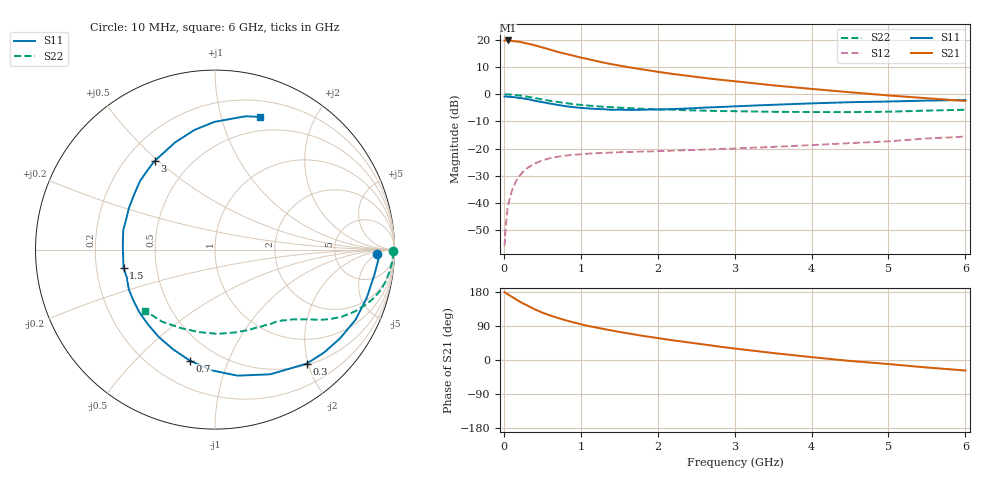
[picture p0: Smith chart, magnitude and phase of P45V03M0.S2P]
! SIEMENS Small Signal Semiconductors
! BFP182
! Si NPN RF Bipolar Junction Transistor in SOT143
! VCE = 5 V  IC = 3 mA
! Common Emitter S-Parameters:  March  1996
# GHz  S  MA  R  50
!  f  S11  S21  S12  S22
! GHz  MAG  ANG  MAG  ANG  MAG  ANG  MAG  ANG
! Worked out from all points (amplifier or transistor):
!   36 points, 10 MHz to 6 GHz, reference 50 ohm
!   highest |S21| = 19.8 dB at 50 MHz (marker M1)
!   |S21| within 3 dB of that: start of sweep to 554.6 MHz
!   unconditionally stable (mu >= 1): 1.952 GHz to 5.777 GHz
!   at 250 MHz: K = 0.16, MSG = 23.8 dB, |S12| = -28.6 dB
!   at 1.4 GHz: K = 0.78, MSG = 16.3 dB, |S12| = -21.5 dB
!   at 6 GHz: K = 0.97, MSG = 6.5 dB, |S12| = -15.6 dB
!   S11 on the Smith chart (normalised r, x): 10 MHz: 18, -5; 300 MHz: 0.52, -1.98; 700 MHz: 0.36, -0.74; 1.5 GHz: 0.32, -0.09; 3 GHz: 0.32, +0.49; 6 GHz: 0.35, +1.34
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0.01  0.9033 -1.7  9.7 178.9  0.0016 80.0  0.9938 -0.6
0.02  0.9118 -3.6  9.732 177.9  0.003 84.9  0.9916 -1.4
0.05  0.8987 -9.1  9.733 173.6  0.0085 85.9  0.991 -3.6
0.1  0.887 -17.7  9.541 167.4  0.0161 78.2  0.9799 -7.2
0.2  0.8541 -35.5  9.235 155.0  0.0311 69.9  0.9497 -13.8
0.25  0.8356 -43.3  8.881 149.3  0.0373 65.5  0.9261 -16.8
0.3  0.8154 -51.2  8.576 144.4  0.0433 62.1  0.9019 -19.4
0.4  0.76 -66.1  7.947 133.8  0.0531 55.2  0.8506 -24.0
0.5  0.7132 -79.9  7.241 125.1  0.0603 48.8  0.8007 -27.8
0.6  0.673 -91.7  6.612 117.7  0.0665 43.9  0.7569 -30.6
0.7  0.6344 -102.7  6 111.1  0.0707 40.1  0.7204 -32.8
0.8  0.6019 -113.1  5.542 104.9  0.074 36.6  0.6864 -34.7
0.9  0.5787 -122.8  5.123 99.6  0.077 34.1  0.6586 -36.2
1.1  0.5467 -140.6  4.403 89.7  0.0807 30.0  0.6162 -39.1
1.5  0.5196 -168.6  3.365 74.1  0.0855 25.1  0.565 -43.9
1.8  0.5167 172.9  2.859 63.9  0.0879 24.1  0.5383 -47.5
2.2  0.5327 154.1  2.354 51.9  0.0914 22.7  0.5175 -53.2
3  0.5976 124.3  1.731 30.3  0.1002 22.3  0.4864 -66.9
3.5  0.6381 110.2  1.455 18.4  0.1073 22.2  0.4743 -76.9
4.5  0.7119 90.2  1.085 -2.5  0.1258 21.0  0.468 -100.7
5.5  0.7622 77.1  0.842 -19.8  0.1531 18.5  0.4981 -126.2
6  0.7813 71.1  0.75 -27.7  0.1662 15.0  0.5171 -138.7
